(* Logix 5000 AddOnInstructionDefinition export NTEC_MAM; software revision ? *)

TYPE NTEC_Axis :   // NTEC Axis:
STRUCT
   StatDriveCommsOK : BOOL;   // Drive is communicating over ENET IP
   StatServoActionStatus : BOOL;   // Motion is enabled and holding position under power.
   StatDriveWarning : BOOL;   // Drive has a Warning
   StatDriveFault : BOOL;   // Drive is Faulted
   StatMotion_AtTarget : BOOL;   // Motion Target Reached
   StatMotion_FollowingError : BOOL;   // Following Error Fault
   StatMotion_LimitExceeded : BOOL;   // Speed or Position Limit Exceeded
   StatMotion_Halt : BOOL;   // Motor is in Halt, still powered on
   StatQuckStop : BOOL;   // Motor is powered off in Quick Stop
   StatMotion_Homed : BOOL;   // Motion Coordinate System Homed
   StatNewCmdToggle : BOOL;   // Bit toggles after new command accepted
   StatCommandError : BOOL;   // Last Command has an Error
   StatCommandErrorCode : DINT;   // Command Error Code
   StatDriveFaultCode : DINT;   // Drive Fault Code
   StatDriveWarningCode : DINT;   // Drive Warning Code
   StatResettingFault : BOOL;   // In fault reset sequence
   StatReadResponse : DINT;   // Response from a Read CMD
   CMD_IP : BOOL;   // Command is In Process
   CMD_DN : BOOL;   // Command is Done
   CMD_ERR : BOOL;   // Command Error during Comms send to Drive
   PDI_CMD : NTEC_PDI_CMD;   // Commands from AOIs
   PDI_Status : NTEC_PDI_Status;   // Status from Drive out to AOIs
   DriveLimits : NTEC_LimitsInDrive;   // Limits read from Drive
END_STRUCT
END_TYPE

TYPE NTEC_LimitsInDrive :   // These are the limits read from the Drive
STRUCT
   PositionLimitMin : DINT;   // Minimum Allowed Position Target (607Bh:1)
   PositionLimitMax : DINT;   // Maximum Allowed Position Target (607Bh:2)
   SoftPositionLimitMin : DINT;   // Minimum Allowed Position (607Dh:1)
   SoftPositionLimitMax : DINT;   // Minimum Allowed Position (607Dh:2)
   VelocityLimitMin : DINT;   // Maximum Allowed Velocity Target negative direction
   VelocityLimitMax : DINT;   // Maximum Allowed Velocity Target positive direction (607Fh)
   MotorSpeedMin : DINT;   // Maximum motor speed in negative direction
   MotorSpeedMax : DINT;   // Maximum motor speed setting in positive direction (6080h)
   AccelLimitMax : DINT;   // Maximum Allowed Accel Target (60C5h)
   DecelLimitMax : DINT;   // Maximum Allowed Decel Target (60C6h)
   PositionWindowNeg : DINT;   // Position Window - negative direction for At Target (6067h)
   PositionWindowPos : DINT;   // Position Window -positive direction for At Target (+/- this value) (6067h)
   VelocityWindowNeg : DINT;   // Velocity Window - negative side for At Target (+/- this value) (606Dh)
   VelocityWindowPos : DINT;   // Velocity Window - positive side for At Target (+/- this value) (606Dh)
   TorqueMaxNegDir : DINT;   // Maximum Torque Target negative direction (0.1% of motor rated current 2031h) (6072h)
   TorqueMaxPosDir : DINT;   // Maximum Torque Target positive direction (0.1% of motor rated current 2031h) (6072h)
   CurrentMaxNegDir : DINT;   // Maximum Current Target negative direction (in 0.1% of rated setting 2031h) (6073h)
   CurrentMaxPosDir : DINT;   // Maximum Current Target positive direction (in 0.1% of rated setting 2031h) (6073h)
END_STRUCT
END_TYPE

TYPE NTEC_PDI_CMD :   // PDI Command Bytes
STRUCT
   SetValue1 : DINT;
   SetValue2 : INT;
   SetValue3 : SINT;
   CMD : SINT;
   DigitalOutputs : DINT;
   NanoJ_Input1 : DINT;
   Trig : BOOL;   // Trigger the Command
   Halt : BOOL;   // Command a HALT
   QuickStop : BOOL;   // Command a QuickStop
END_STRUCT
END_TYPE

TYPE NTEC_PDI_Status :   // PDI Status Bytes
STRUCT
   Status : INT;
   ErrorCode : INT;
   ReturnValue : DINT;
   PositionActualValue : DINT;
   VelocityActualValue : DINT;
   DigitalInputs : DINT;
   TorqueActualValue : INT;
   AnalogInput1 : INT;
   FollowingError : DINT;
   NanoJ_Output1 : DINT;
END_STRUCT
END_TYPE

ADD_ON_INSTRUCTION NTEC_WRITE   (* revision 1.6, vendor Third Coast Automation, Nashville, TN, ExecutePrescan, ExecuteEnableInFalse *)
// WRITE instruction writes the value entered into the AOI, into the specified object in the Drive.  Enter the target object's index and sub-index (typically 16#xxxx hex values).
// Revision note:
// Release Aug 27, 2024, update CPS instructions LEN
// Help:
// AOI written by:
// Tim Cochran
// Third Coast Automation
// Nashville, TN
// MAS ERR_Codes:
// 2: Input parameter range error – review and fix input parameters.
// 3: Command Error response from the Drive after command sent.
// 10: Communications Failed to Drive.
// 11: Drive Fault during this AOIs command sequence.
// 12: Quick Stop triggered by software outside of this AOI.
// 13: Command Error response from the Drive.
// 14: Enable input changed to False during sequence due to Drive Fault or Offline.
VAR_IN_OUT
   NTEC_Axis : NTEC_Axis; {required}   // NTEC Axis Tag
END_VAR
VAR_INPUT
   Index : DINT; {required}   // Index
   SubIndex : DINT; {required}   // Sub-Index
END_VAR
VAR_OUTPUT
   EN : BOOL; {visible}   // Enabled
   DN : BOOL; {visible}   // Successfully Done
END_VAR
VAR_INPUT
   Value : DINT; {required}   // WriteValue
END_VAR
VAR_OUTPUT
   ERR : BOOL; {visible}   // Instruction Error
   ERR_Code : DINT; {access Read Only, visible}   // Instruction Error Code
END_VAR
VAR
   State : DINT; {access None}
   Enable : BOOL; {access None}
   InputRangesOK : BOOL; {access None}
   local_SubIndex : DINT; {access None}
   local_Index : DINT; {access None}
   tmr_Verify : TIMER; {access None}
   local_Value : DINT; {access None}
END_VAR

ROUTINE EnableInFalse   (* ladder *)
// Enable In False Routine
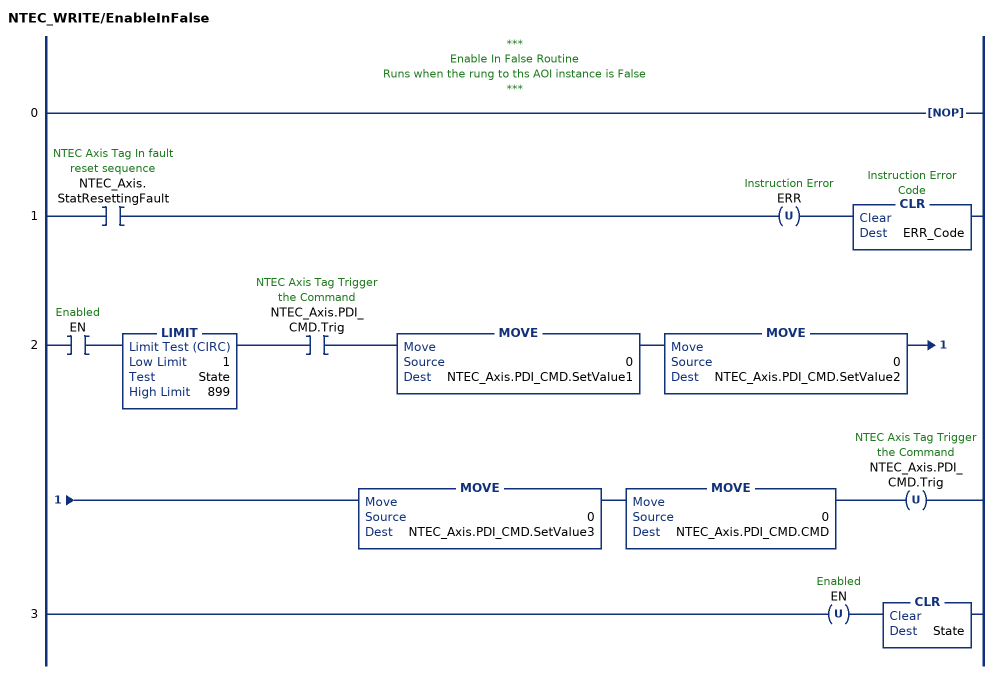
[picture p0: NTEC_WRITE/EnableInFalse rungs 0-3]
   // ***
   // Enable In False Routine
   // Runs when the rung to ths AOI instance is False
   // ***
   0: NOP();
   1: XIC(NTEC_Axis.StatResettingFault)OTU(ERR)CLR(ERR_Code);
   2: XIC(EN)LIMIT(1,State,899)XIC(NTEC_Axis.PDI_CMD.Trig)MOVE(0,NTEC_Axis.PDI_CMD.SetValue1)MOVE(0,NTEC_Axis.PDI_CMD.SetValue2)MOVE(0,NTEC_Axis.PDI_CMD.SetValue3)MOVE(0,NTEC_Axis.PDI_CMD.CMD)OTU(NTEC_Axis.PDI_CMD.Trig);
   3: OTU(EN)CLR(State);
END_ROUTINE

ROUTINE Logic   (* ladder *)
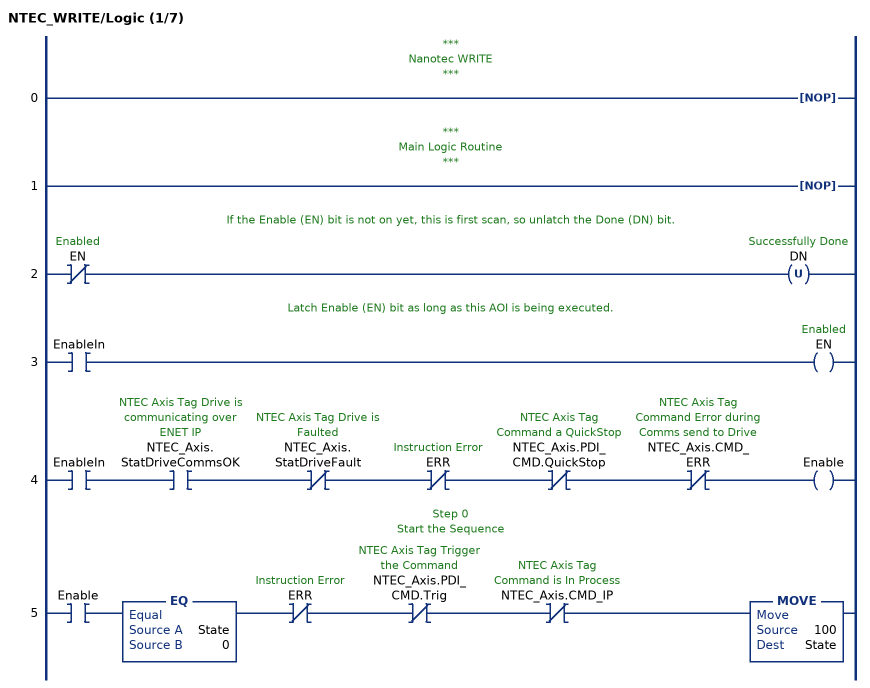
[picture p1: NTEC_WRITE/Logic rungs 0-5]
   // ***
   // Nanotec WRITE
   // ***
   0: NOP();
   // ***
   // Main Logic Routine
   // ***
   1: NOP();
   // If the Enable (EN) bit is not on yet, this is first scan, so unlatch the Done (DN) bit.
   2: XIO(EN)OTU(DN);
   // Latch Enable (EN) bit as long as this AOI is being executed.
   3: XIC(EnableIn)OTE(EN);
   4: XIC(EnableIn)XIC(NTEC_Axis.StatDriveCommsOK)XIO(NTEC_Axis.StatDriveFault)XIO(ERR)XIO(NTEC_Axis.PDI_CMD.QuickStop)XIO(NTEC_Axis.CMD_ERR)OTE(Enable);
   // Step 0
   // Start the Sequence
   5: XIC(Enable)EQ(State,0)XIO(ERR)XIO(NTEC_Axis.PDI_CMD.Trig)XIO(NTEC_Axis.CMD_IP)MOVE(100,State);
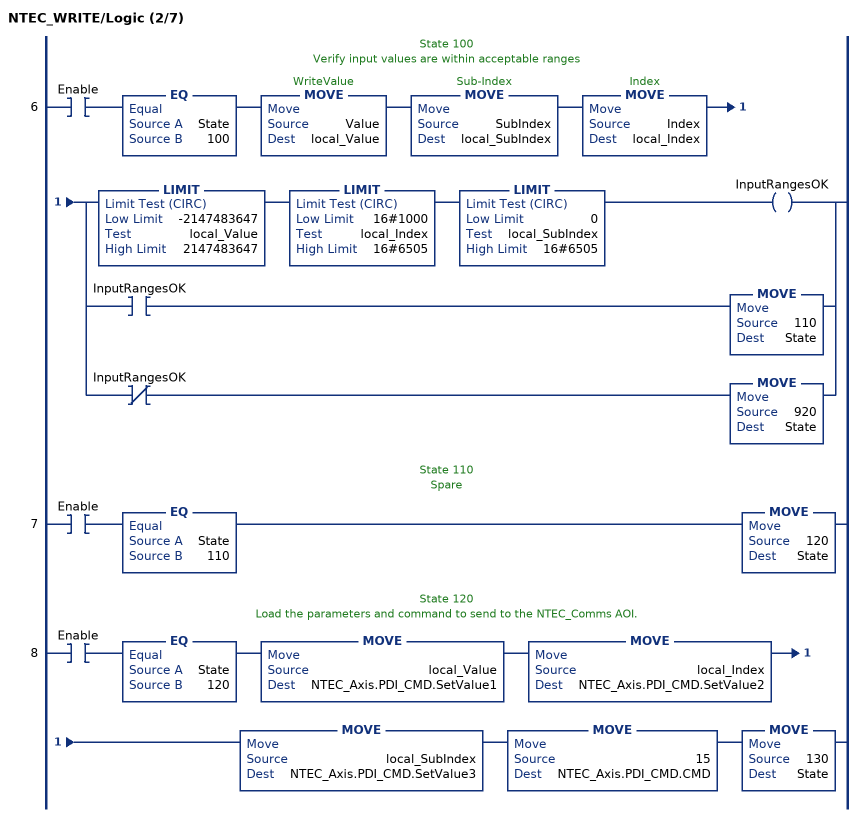
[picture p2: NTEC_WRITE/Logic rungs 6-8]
   // State 100
   // Verify input values are within acceptable ranges
   6: XIC(Enable)EQ(State,100)MOVE(Value,local_Value)MOVE(SubIndex,local_SubIndex)MOVE(Index,local_Index)[LIMIT(-2147483647,local_Value,2147483647) LIMIT(16#1000,local_Index,16#6505) LIMIT(0,local_SubIndex,16#6505) OTE(InputRangesOK) ,XIC(InputRangesOK) MOVE(110,State) ,XIO(InputRangesOK) MOVE(920,State) ];
   // State 110
   // Spare
   7: XIC(Enable)EQ(State,110)MOVE(120,State);
   // State 120
   // Load the parameters and command to send to the NTEC_Comms AOI.
   8: XIC(Enable)EQ(State,120)MOVE(local_Value,NTEC_Axis.PDI_CMD.SetValue1)MOVE(local_Index,NTEC_Axis.PDI_CMD.SetValue2)MOVE(local_SubIndex,NTEC_Axis.PDI_CMD.SetValue3)MOVE(15,NTEC_Axis.PDI_CMD.CMD)MOVE(130,State);
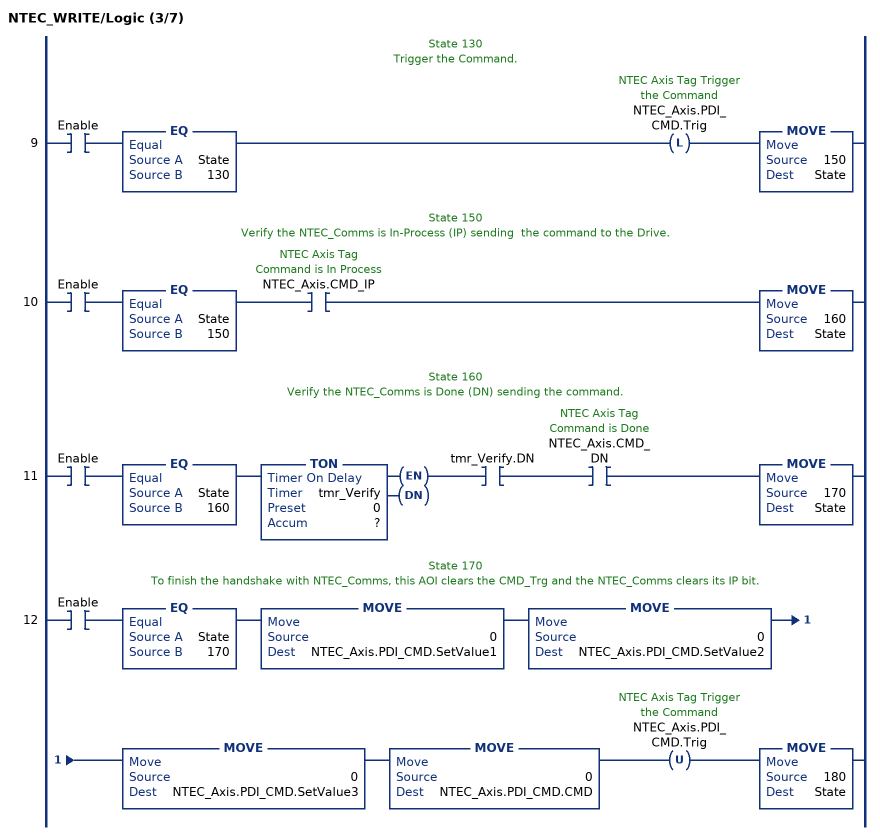
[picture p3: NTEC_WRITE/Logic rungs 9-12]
   // State 130
   // Trigger the Command.
   9: XIC(Enable)EQ(State,130)OTL(NTEC_Axis.PDI_CMD.Trig)MOVE(150,State);
   // State 150
   // Verify the NTEC_Comms is In-Process (IP) sending  the command to the Drive.
   10: XIC(Enable)EQ(State,150)XIC(NTEC_Axis.CMD_IP)MOVE(160,State);
   // State 160
   // Verify the NTEC_Comms is Done (DN) sending the command.
   11: XIC(Enable)EQ(State,160)TON(tmr_Verify,?,?)XIC(tmr_Verify.DN)XIC(NTEC_Axis.CMD_DN)MOVE(170,State);
   // State 170
   // To finish the handshake with NTEC_Comms, this AOI clears the CMD_Trg and the NTEC_Comms clears its IP bit.
   12: XIC(Enable)EQ(State,170)MOVE(0,NTEC_Axis.PDI_CMD.SetValue1)MOVE(0,NTEC_Axis.PDI_CMD.SetValue2)MOVE(0,NTEC_Axis.PDI_CMD.SetValue3)MOVE(0,NTEC_Axis.PDI_CMD.CMD)OTU(NTEC_Axis.PDI_CMD.Trig)MOVE(180,State);
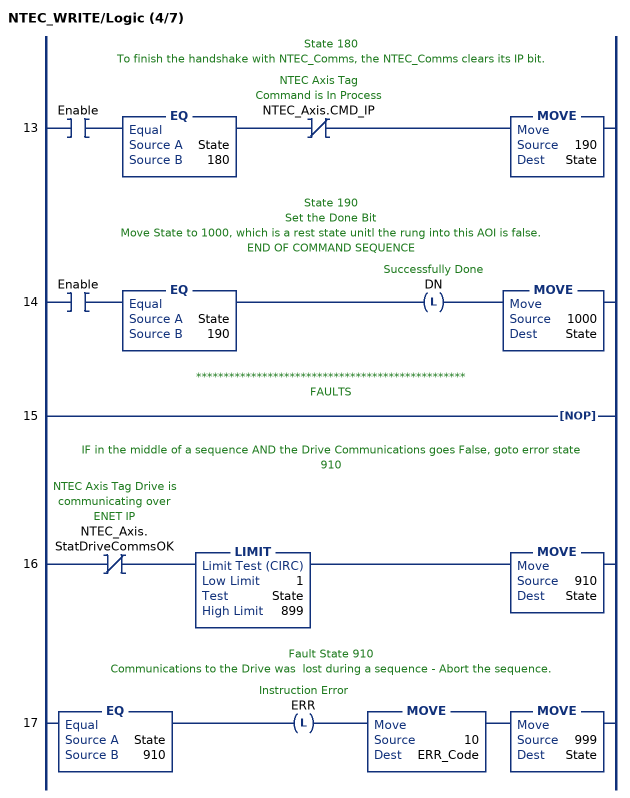
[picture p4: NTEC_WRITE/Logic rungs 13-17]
   // State 180
   // To finish the handshake with NTEC_Comms, the NTEC_Comms clears its IP bit.
   13: XIC(Enable)EQ(State,180)XIO(NTEC_Axis.CMD_IP)MOVE(190,State);
   // State 190
   // Set the Done Bit
   // Move State to 1000, which is a rest state unitl the rung into this AOI is false.
   // END OF COMMAND SEQUENCE
   14: XIC(Enable)EQ(State,190)OTL(DN)MOVE(1000,State);
   // *************************************************
   // FAULTS
   15: NOP();
   // IF in the middle of a sequence AND the Drive Communications goes False, goto error state 910
   16: XIO(NTEC_Axis.StatDriveCommsOK)LIMIT(1,State,899)MOVE(910,State);
   // Fault State 910
   // Communications to the Drive was  lost during a sequence - Abort the sequence.
   17: EQ(State,910)OTL(ERR)MOVE(10,ERR_Code)MOVE(999,State);
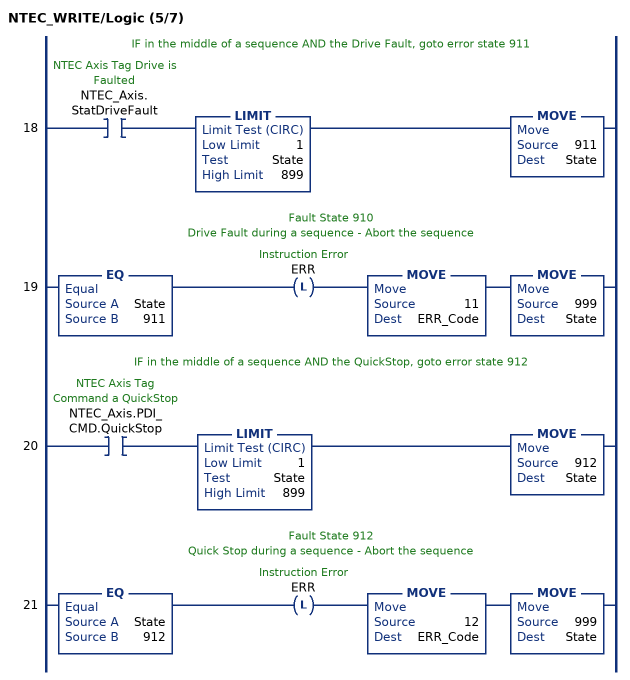
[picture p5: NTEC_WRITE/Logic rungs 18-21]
   // IF in the middle of a sequence AND the Drive Fault, goto error state 911
   18: XIC(NTEC_Axis.StatDriveFault)LIMIT(1,State,899)MOVE(911,State);
   // Fault State 910
   // Drive Fault during a sequence - Abort the sequence
   19: EQ(State,911)OTL(ERR)MOVE(11,ERR_Code)MOVE(999,State);
   // IF in the middle of a sequence AND the QuickStop, goto error state 912
   20: XIC(NTEC_Axis.PDI_CMD.QuickStop)LIMIT(1,State,899)MOVE(912,State);
   // Fault State 912
   // Quick Stop during a sequence - Abort the sequence
   21: EQ(State,912)OTL(ERR)MOVE(12,ERR_Code)MOVE(999,State);
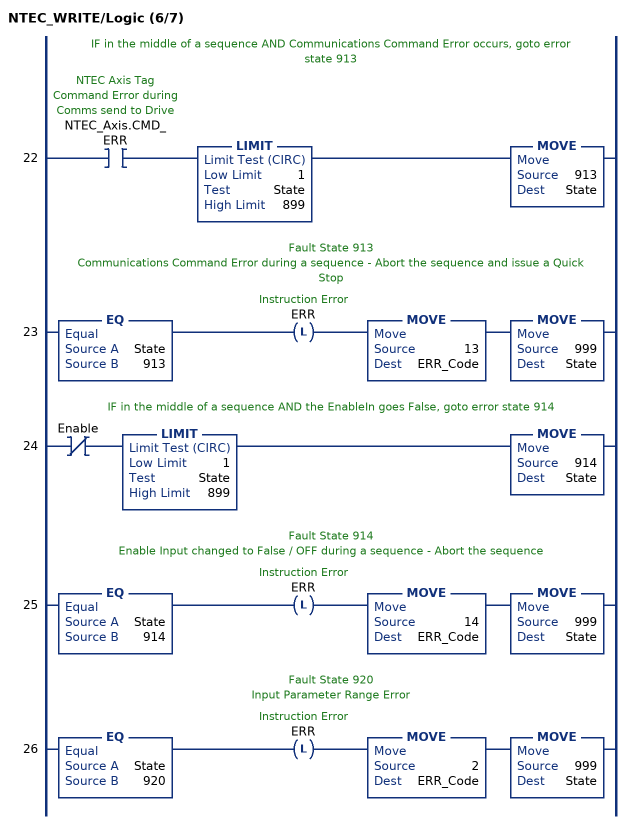
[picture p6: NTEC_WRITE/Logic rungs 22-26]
   // IF in the middle of a sequence AND Communications Command Error occurs, goto error state 913
   22: XIC(NTEC_Axis.CMD_ERR)LIMIT(1,State,899)MOVE(913,State);
   // Fault State 913
   // Communications Command Error during a sequence - Abort the sequence and issue a Quick Stop
   23: EQ(State,913)OTL(ERR)MOVE(13,ERR_Code)MOVE(999,State);
   // IF in the middle of a sequence AND the EnableIn goes False, goto error state 914
   24: XIO(Enable)LIMIT(1,State,899)MOVE(914,State);
   // Fault State 914
   // Enable Input changed to False / OFF during a sequence - Abort the sequence
   25: EQ(State,914)OTL(ERR)MOVE(14,ERR_Code)MOVE(999,State);
   // Fault State 920
   // Input Parameter Range Error
   26: EQ(State,920)OTL(ERR)MOVE(2,ERR_Code)MOVE(999,State);
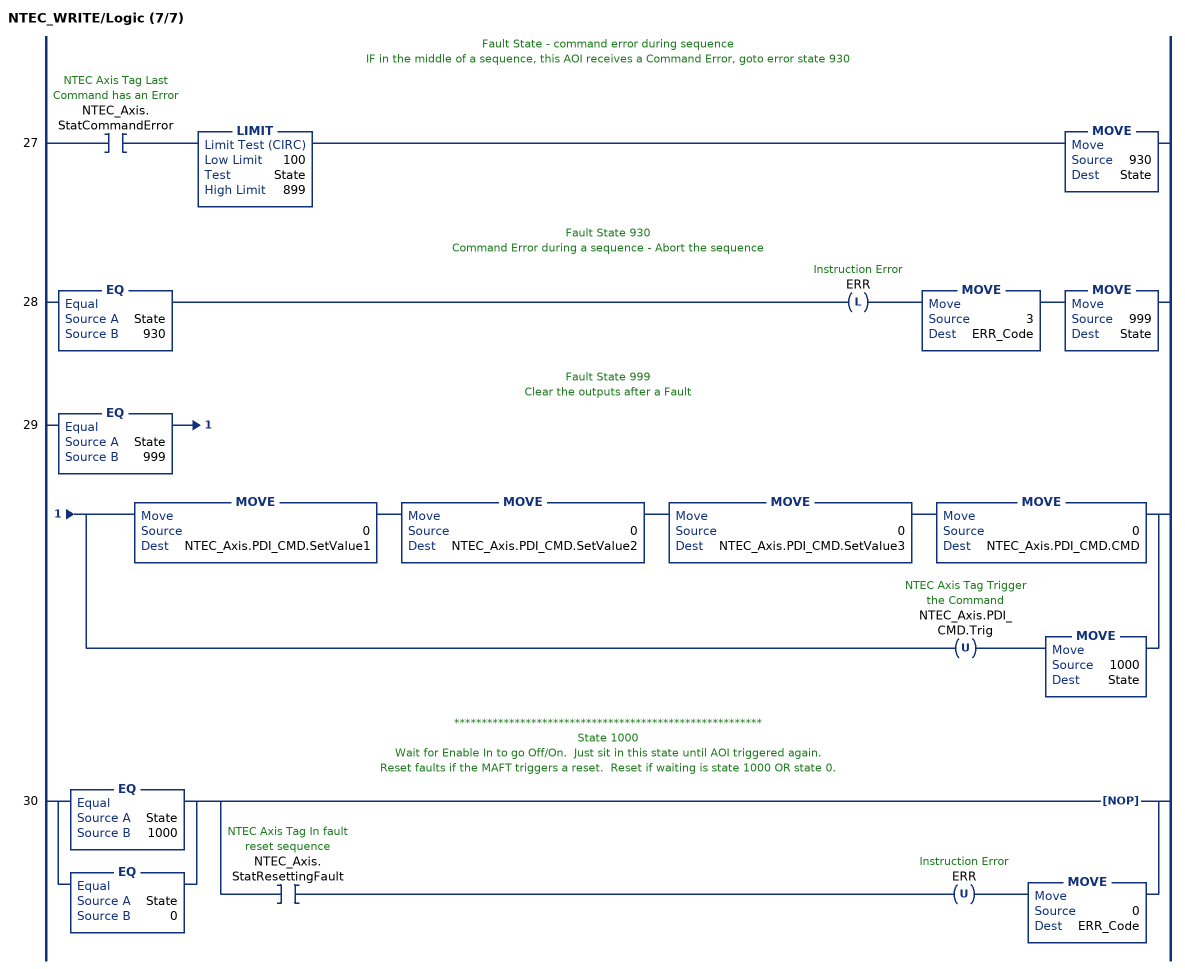
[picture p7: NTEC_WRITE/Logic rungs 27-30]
   // Fault State - command error during sequence
   // IF in the middle of a sequence, this AOI receives a Command Error, goto error state 930
   27: XIC(NTEC_Axis.StatCommandError)LIMIT(100,State,899)MOVE(930,State);
   // Fault State 930
   // Command Error during a sequence - Abort the sequence
   28: EQ(State,930)OTL(ERR)MOVE(3,ERR_Code)MOVE(999,State);
   // Fault State 999
   // Clear the outputs after a Fault
   29: EQ(State,999)[MOVE(0,NTEC_Axis.PDI_CMD.SetValue1) MOVE(0,NTEC_Axis.PDI_CMD.SetValue2) MOVE(0,NTEC_Axis.PDI_CMD.SetValue3) MOVE(0,NTEC_Axis.PDI_CMD.CMD) ,OTU(NTEC_Axis.PDI_CMD.Trig) MOVE(1000,State) ];
   // ********************************************************
   // State 1000
   // Wait for Enable In to go Off/On.  Just sit in this state until AOI triggered again.
   // Reset faults if the MAFT triggers a reset.  Reset if waiting is state 1000 OR state 0.
   30: [EQ(State,1000) ,EQ(State,0) ][NOP() ,XIC(NTEC_Axis.StatResettingFault) OTU(ERR) MOVE(0,ERR_Code) ];
END_ROUTINE

ROUTINE Postscan   (* ladder *)
// Home Post-Scan Routine
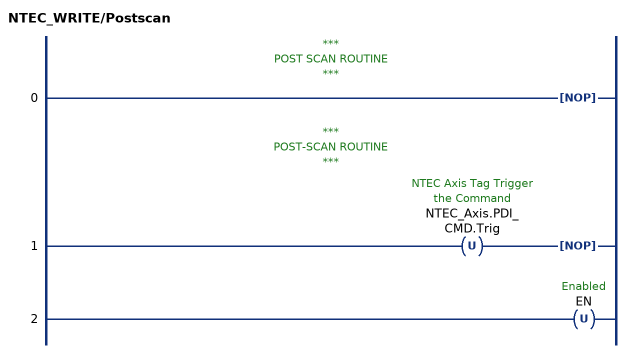
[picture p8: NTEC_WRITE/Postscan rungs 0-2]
   // ***
   // POST SCAN ROUTINE
   // ***
   0: NOP();
   // ***
   // POST-SCAN ROUTINE
   // ***
   1: OTU(NTEC_Axis.PDI_CMD.Trig)NOP();
   2: OTU(EN);
END_ROUTINE

ROUTINE Prescan   (* ladder *)
// Home Pre-Scan Routine
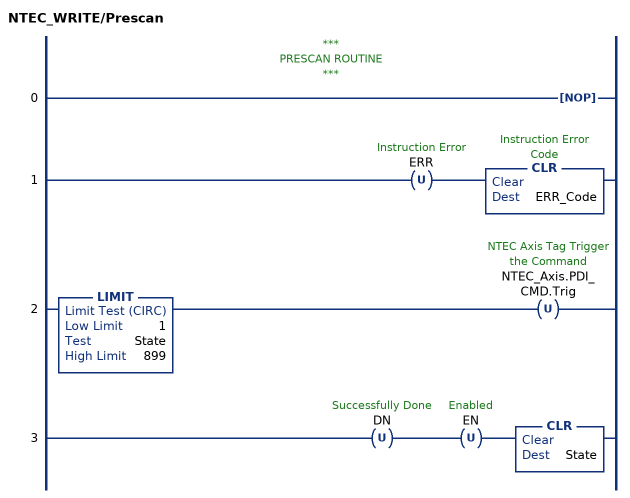
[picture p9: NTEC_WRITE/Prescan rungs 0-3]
   // ***
   // PRESCAN ROUTINE
   // ***
   0: NOP();
   1: OTU(ERR)CLR(ERR_Code);
   2: LIMIT(1,State,899)OTU(NTEC_Axis.PDI_CMD.Trig);
   3: OTU(DN)OTU(EN)CLR(State);
END_ROUTINE
END_ADD_ON_INSTRUCTION

ADD_ON_INSTRUCTION NTEC_MAM   (* revision 1.6, vendor Third Coast Automation, Nashville, TN, ExecutePrescan, ExecuteEnableInFalse *)
// Motion Axis Move (MAM)
// Move the servo axis to a target position.
// Move Type:
// 1=Absolute
// 2=Incremental (Relative)
// All input parameters are entered into the AOI in whole numbers, in the units as setup and scaled in the Drive.
// Revision note:
// Release Aug 27, 2024, update CPS instructions LEN
// Help:
// AOI written by:
// Tim Cochran
// Third Coast Automation
// Nashville, TN
// MAM ERR_Codes:
// 2: Input parameter range error – review and fix input parameters.
// 3: Command Error response from the Drive after command sent.
// 4: Command Error after Accel value was sent to the Drive.
// 5: Command Error after Decel value was sent to the Drive.
// 10: Communications Failed to Drive.
// 11: Drive Fault during this AOIs command sequence.
// 12: Quick Stop triggered by software outside of this AOI.
// 13: Command Error response from the Drive.
// 14: Enable input changed to False during sequence due to Drive Fault or Offline.
VAR_IN_OUT
   NTEC_Axis : NTEC_Axis; {required}   // NTEC Axis Tag
END_VAR
VAR_INPUT
   MoveType : DINT; {required}   // 1=Absolute 2= Relative (Incremental)
   Position : DINT; {required}   // Position value for move location
   Velocity : DINT; {required}   // Velocity in Drive units / sec
   Acceleration : DINT; {required}   // Accel in Drive units/sec^2
   Deceleration : DINT; {required}   // Decel in Drive units/sec^2
END_VAR
VAR_OUTPUT
   EN : BOOL; {access Read Only, visible}   // Enabled
   IP : BOOL; {visible}   // In Process
   DN : BOOL; {visible}   // Successfully Done
   ERR : BOOL; {visible}   // Instruction Error
   ERR_Code : DINT; {access Read Only, visible}   // Instruction Error Code
END_VAR
VAR
   State : DINT; {access None}
   Enable : BOOL; {access None}
   local_MoveType : DINT := 2; {access None}
   local_Position : DINT; {access None}
   local_Acceleration : DINT; {access None}
   InputRangesOK : BOOL; {access None}
   tmr_Verify : TIMER := (PRE := 20); {access None}
   local_Deceleration : DINT; {access None}
   local_Velocity : INT; {access None}
   Write1_cntrl : NTEC_WRITE; {access None}
   Write2_cntrl : NTEC_WRITE; {access None}
   MoveStarted : BOOL; {access None}
   MovePositionDelta : DINT; {access None}
   LowLimitPositionWindow : DINT := -50; {access None}
   HighLimitPositionWindow : DINT := 50; {access None}
END_VAR

ROUTINE EnableInFalse   (* ladder *)
// Enable In False Routine
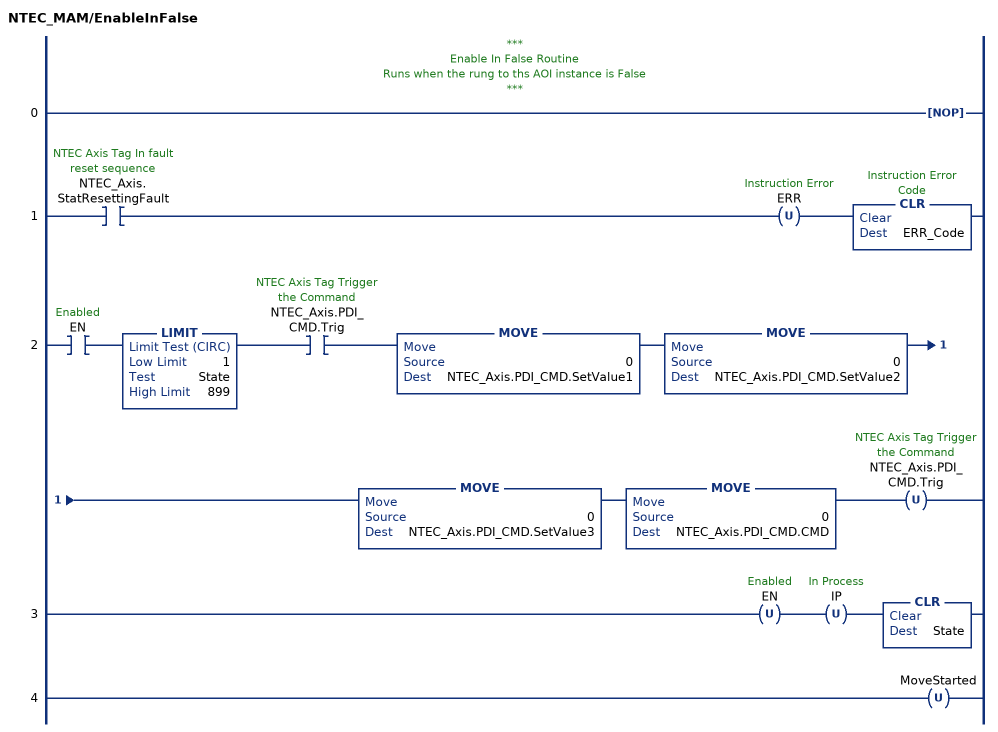
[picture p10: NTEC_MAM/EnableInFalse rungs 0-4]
   // ***
   // Enable In False Routine
   // Runs when the rung to ths AOI instance is False
   // ***
   0: NOP();
   1: XIC(NTEC_Axis.StatResettingFault)OTU(ERR)CLR(ERR_Code);
   2: XIC(EN)LIMIT(1,State,899)XIC(NTEC_Axis.PDI_CMD.Trig)MOVE(0,NTEC_Axis.PDI_CMD.SetValue1)MOVE(0,NTEC_Axis.PDI_CMD.SetValue2)MOVE(0,NTEC_Axis.PDI_CMD.SetValue3)MOVE(0,NTEC_Axis.PDI_CMD.CMD)OTU(NTEC_Axis.PDI_CMD.Trig);
   3: OTU(EN)OTU(IP)CLR(State);
   4: OTU(MoveStarted);
END_ROUTINE

ROUTINE Logic   (* ladder *)
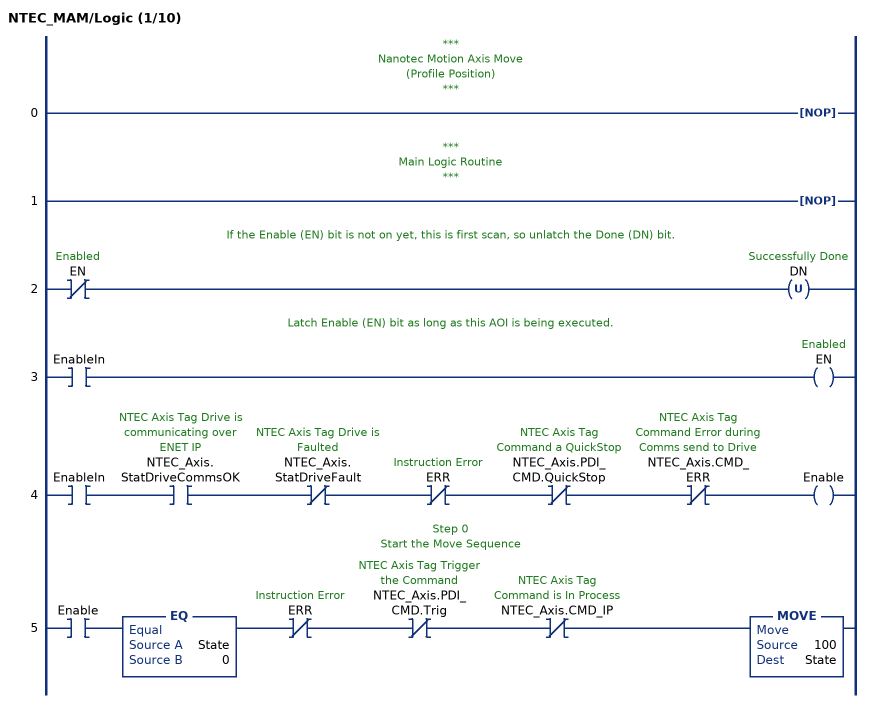
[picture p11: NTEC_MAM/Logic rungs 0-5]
   // ***
   // Nanotec Motion Axis Move
   // (Profile Position)
   // ***
   0: NOP();
   // ***
   // Main Logic Routine
   // ***
   1: NOP();
   // If the Enable (EN) bit is not on yet, this is first scan, so unlatch the Done (DN) bit.
   2: XIO(EN)OTU(DN);
   // Latch Enable (EN) bit as long as this AOI is being executed.
   3: XIC(EnableIn)OTE(EN);
   4: XIC(EnableIn)XIC(NTEC_Axis.StatDriveCommsOK)XIO(NTEC_Axis.StatDriveFault)XIO(ERR)XIO(NTEC_Axis.PDI_CMD.QuickStop)XIO(NTEC_Axis.CMD_ERR)OTE(Enable);
   // Step 0
   // Start the Move Sequence
   5: XIC(Enable)EQ(State,0)XIO(ERR)XIO(NTEC_Axis.PDI_CMD.Trig)XIO(NTEC_Axis.CMD_IP)MOVE(100,State);
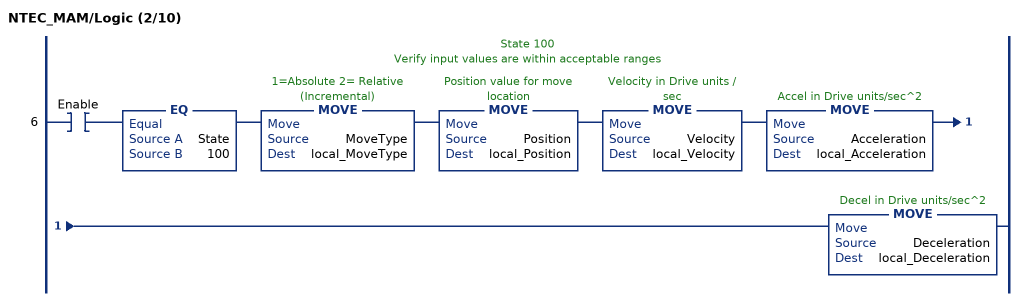
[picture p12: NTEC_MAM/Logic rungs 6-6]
   // State 100
   // Verify input values are within acceptable ranges
   6: XIC(Enable)EQ(State,100)MOVE(MoveType,local_MoveType)MOVE(Position,local_Position)MOVE(Velocity,local_Velocity)MOVE(Acceleration,local_Acceleration)MOVE(Deceleration,local_Deceleration);
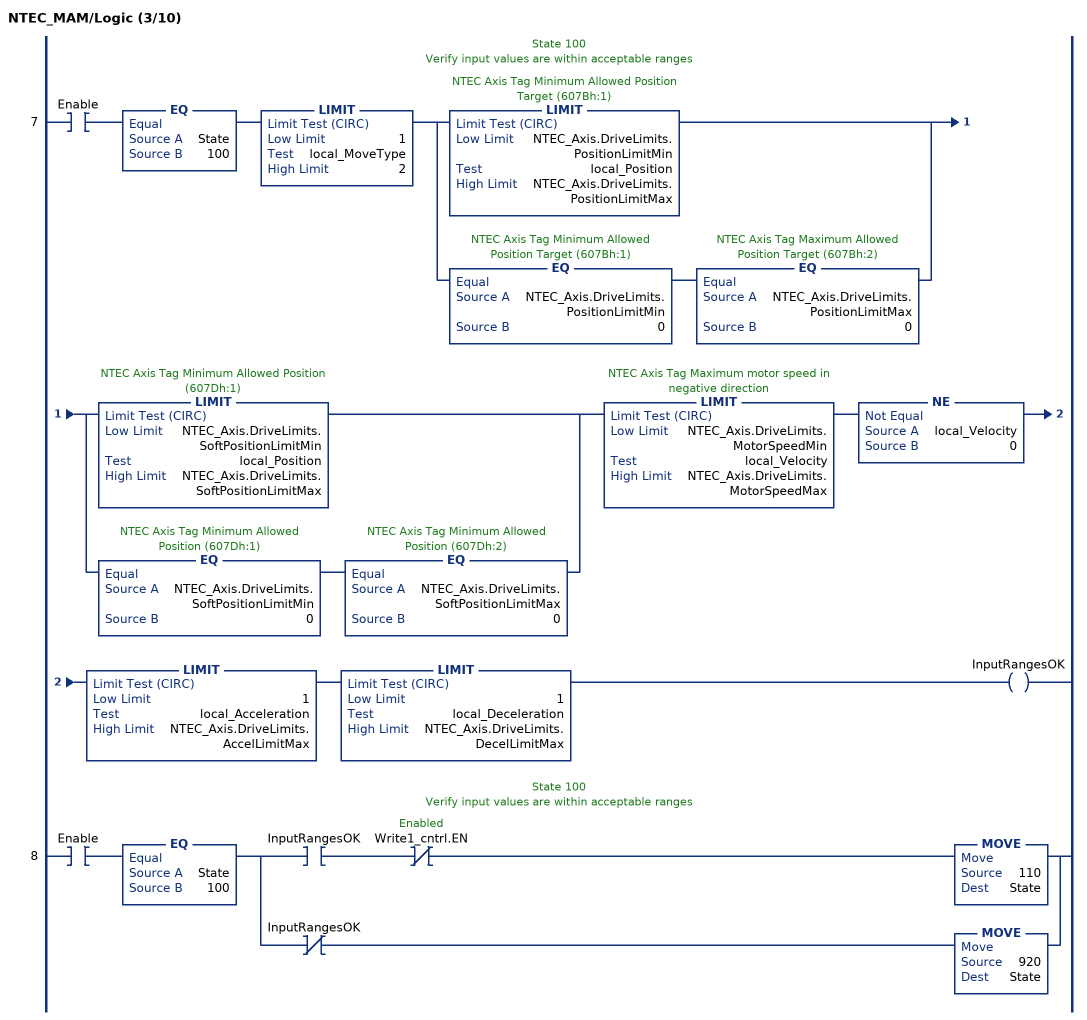
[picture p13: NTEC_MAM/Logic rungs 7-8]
   // State 100
   // Verify input values are within acceptable ranges
   7: XIC(Enable)EQ(State,100)LIMIT(1,local_MoveType,2)[LIMIT(NTEC_Axis.DriveLimits.PositionLimitMin,local_Position,NTEC_Axis.DriveLimits.PositionLimitMax) ,EQ(NTEC_Axis.DriveLimits.PositionLimitMin,0) EQ(NTEC_Axis.DriveLimits.PositionLimitMax,0) ][LIMIT(NTEC_Axis.DriveLimits.SoftPositionLimitMin,local_Position,NTEC_Axis.DriveLimits.SoftPositionLimitMax) ,EQ(NTEC_Axis.DriveLimits.SoftPositionLimitMin,0) EQ(NTEC_Axis.DriveLimits.SoftPositionLimitMax,0) ]LIMIT(NTEC_Axis.DriveLimits.MotorSpeedMin,local_Velocity,NTEC_Axis.DriveLimits.MotorSpeedMax)NE(local_Velocity,0)LIMIT(1,local_Acceleration,NTEC_Axis.DriveLimits.AccelLimitMax)LIMIT(1,local_Deceleration,NTEC_Axis.DriveLimits.DecelLimitMax)OTE(InputRangesOK);
   // State 100
   // Verify input values are within acceptable ranges
   8: XIC(Enable)EQ(State,100)[XIC(InputRangesOK) XIO(Write1_cntrl.EN) MOVE(110,State) ,XIO(InputRangesOK) MOVE(920,State) ];
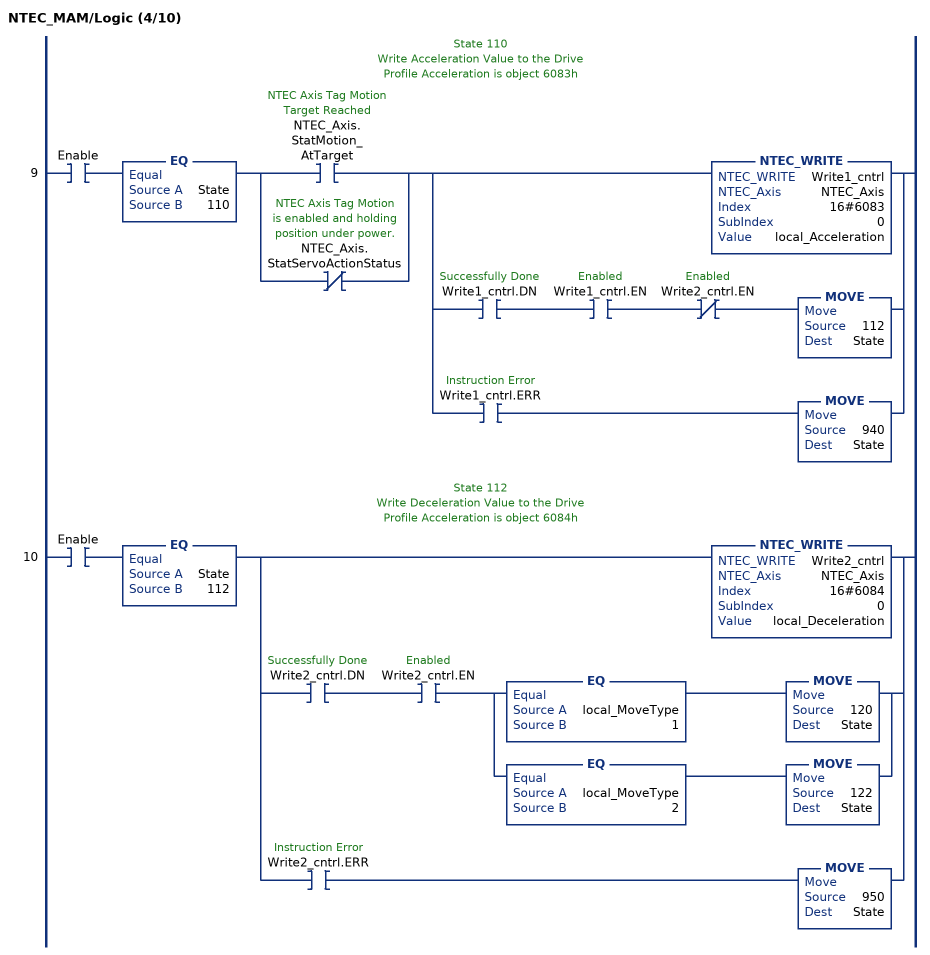
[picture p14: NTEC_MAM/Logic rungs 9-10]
   // State 110
   // Write Acceleration Value to the Drive
   // Profile Acceleration is object 6083h
   9: XIC(Enable)EQ(State,110)[XIC(NTEC_Axis.StatMotion_AtTarget) ,XIO(NTEC_Axis.StatServoActionStatus) ][NTEC_WRITE(Write1_cntrl,NTEC_Axis,16#6083,0,local_Acceleration) ,XIC(Write1_cntrl.DN) XIC(Write1_cntrl.EN) XIO(Write2_cntrl.EN) MOVE(112,State) ,XIC(Write1_cntrl.ERR) MOVE(940,State) ];
   // State 112
   // Write Deceleration Value to the Drive
   // Profile Acceleration is object 6084h
   10: XIC(Enable)EQ(State,112)[NTEC_WRITE(Write2_cntrl,NTEC_Axis,16#6084,0,local_Deceleration) ,XIC(Write2_cntrl.DN) XIC(Write2_cntrl.EN) [EQ(local_MoveType,1) MOVE(120,State) ,EQ(local_MoveType,2) MOVE(122,State) ] ,XIC(Write2_cntrl.ERR) MOVE(950,State) ];
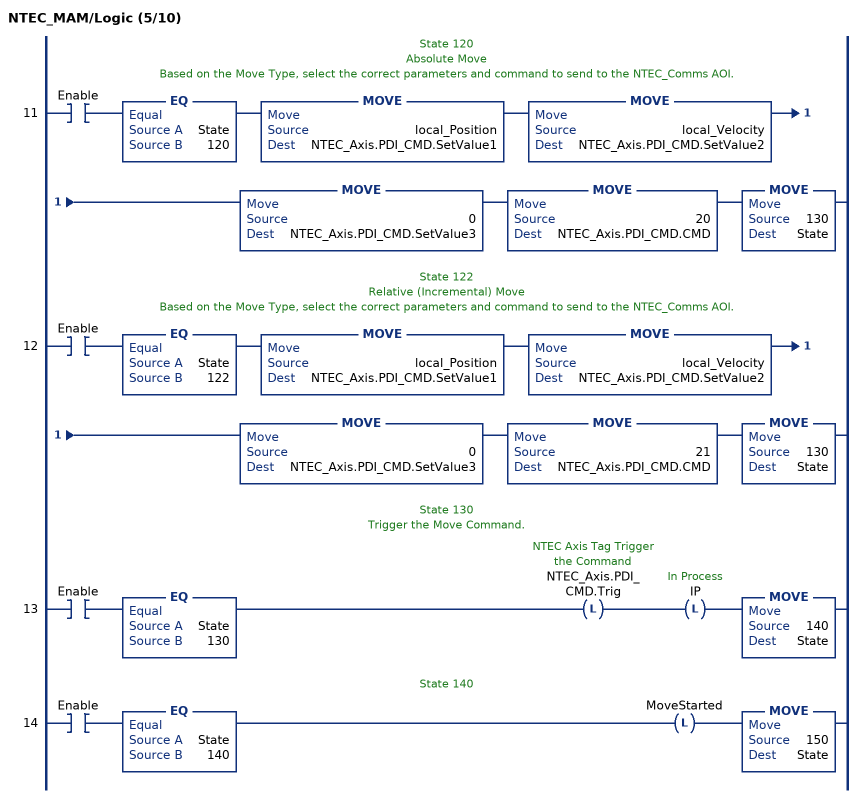
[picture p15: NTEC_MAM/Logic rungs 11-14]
   // State 120
   // Absolute Move
   // Based on the Move Type, select the correct parameters and command to send to the NTEC_Comms AOI.
   11: XIC(Enable)EQ(State,120)MOVE(local_Position,NTEC_Axis.PDI_CMD.SetValue1)MOVE(local_Velocity,NTEC_Axis.PDI_CMD.SetValue2)MOVE(0,NTEC_Axis.PDI_CMD.SetValue3)MOVE(20,NTEC_Axis.PDI_CMD.CMD)MOVE(130,State);
   // State 122
   // Relative (Incremental) Move
   // Based on the Move Type, select the correct parameters and command to send to the NTEC_Comms AOI.
   12: XIC(Enable)EQ(State,122)MOVE(local_Position,NTEC_Axis.PDI_CMD.SetValue1)MOVE(local_Velocity,NTEC_Axis.PDI_CMD.SetValue2)MOVE(0,NTEC_Axis.PDI_CMD.SetValue3)MOVE(21,NTEC_Axis.PDI_CMD.CMD)MOVE(130,State);
   // State 130
   // Trigger the Move Command.
   13: XIC(Enable)EQ(State,130)OTL(NTEC_Axis.PDI_CMD.Trig)OTL(IP)MOVE(140,State);
   // State 140
   14: XIC(Enable)EQ(State,140)OTL(MoveStarted)MOVE(150,State);
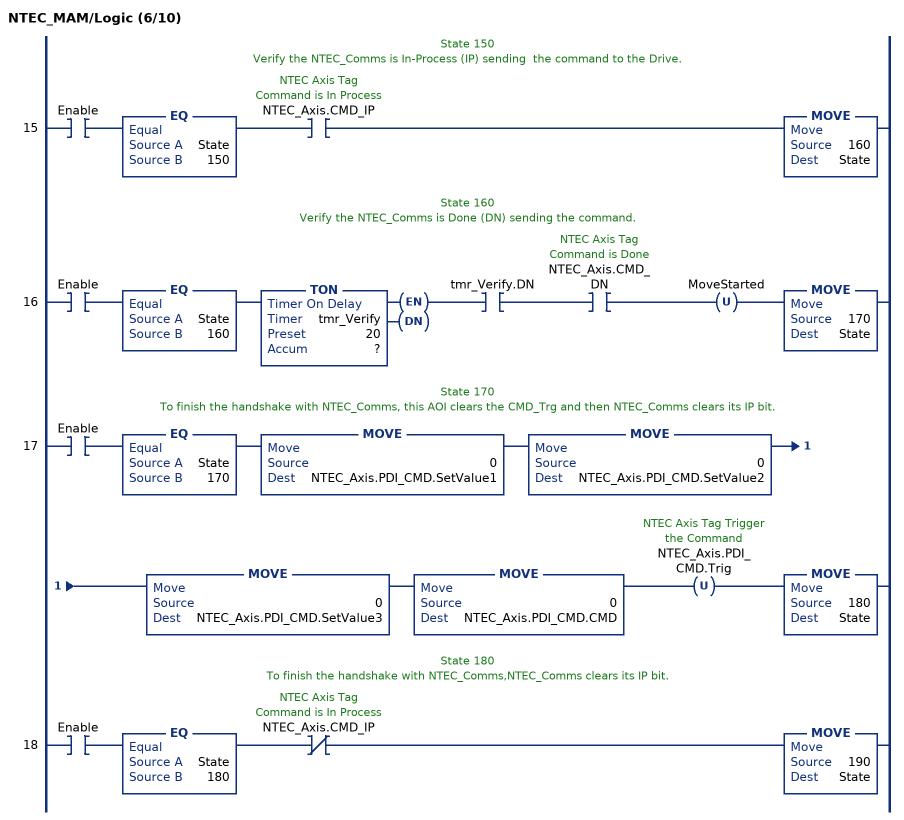
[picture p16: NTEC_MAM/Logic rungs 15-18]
   // State 150
   // Verify the NTEC_Comms is In-Process (IP) sending  the command to the Drive.
   15: XIC(Enable)EQ(State,150)XIC(NTEC_Axis.CMD_IP)MOVE(160,State);
   // State 160
   // Verify the NTEC_Comms is Done (DN) sending the command.
   16: XIC(Enable)EQ(State,160)TON(tmr_Verify,?,?)XIC(tmr_Verify.DN)XIC(NTEC_Axis.CMD_DN)OTU(MoveStarted)MOVE(170,State);
   // State 170
   // To finish the handshake with NTEC_Comms, this AOI clears the CMD_Trg and then NTEC_Comms clears its IP bit.
   17: XIC(Enable)EQ(State,170)MOVE(0,NTEC_Axis.PDI_CMD.SetValue1)MOVE(0,NTEC_Axis.PDI_CMD.SetValue2)MOVE(0,NTEC_Axis.PDI_CMD.SetValue3)MOVE(0,NTEC_Axis.PDI_CMD.CMD)OTU(NTEC_Axis.PDI_CMD.Trig)MOVE(180,State);
   // State 180
   // To finish the handshake with NTEC_Comms,NTEC_Comms clears its IP bit.
   18: XIC(Enable)EQ(State,180)XIO(NTEC_Axis.CMD_IP)MOVE(190,State);
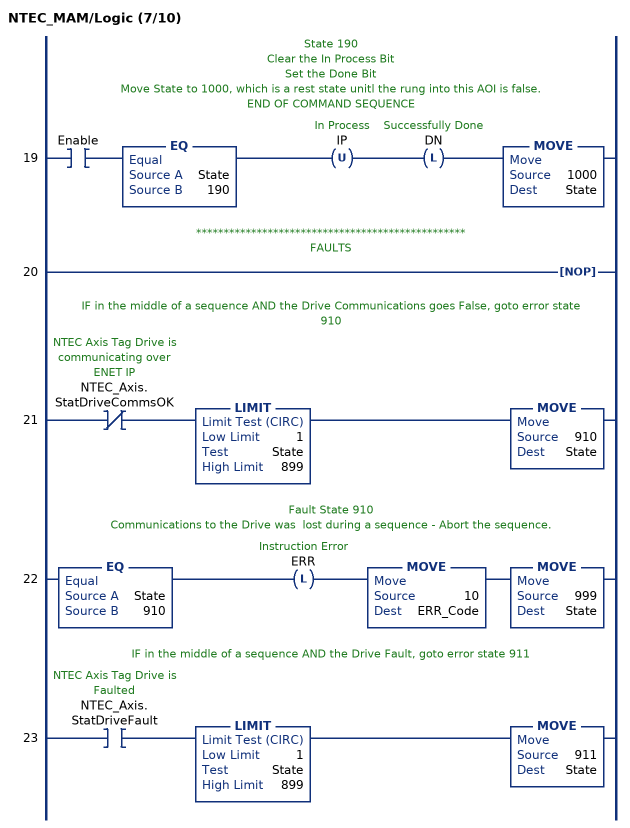
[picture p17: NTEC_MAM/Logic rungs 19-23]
   // State 190
   // Clear the In Process Bit
   // Set the Done Bit
   // Move State to 1000, which is a rest state unitl the rung into this AOI is false.
   // END OF COMMAND SEQUENCE
   19: XIC(Enable)EQ(State,190)OTU(IP)OTL(DN)MOVE(1000,State);
   // *************************************************
   // FAULTS
   20: NOP();
   // IF in the middle of a sequence AND the Drive Communications goes False, goto error state 910
   21: XIO(NTEC_Axis.StatDriveCommsOK)LIMIT(1,State,899)MOVE(910,State);
   // Fault State 910
   // Communications to the Drive was  lost during a sequence - Abort the sequence.
   22: EQ(State,910)OTL(ERR)MOVE(10,ERR_Code)MOVE(999,State);
   // IF in the middle of a sequence AND the Drive Fault, goto error state 911
   23: XIC(NTEC_Axis.StatDriveFault)LIMIT(1,State,899)MOVE(911,State);
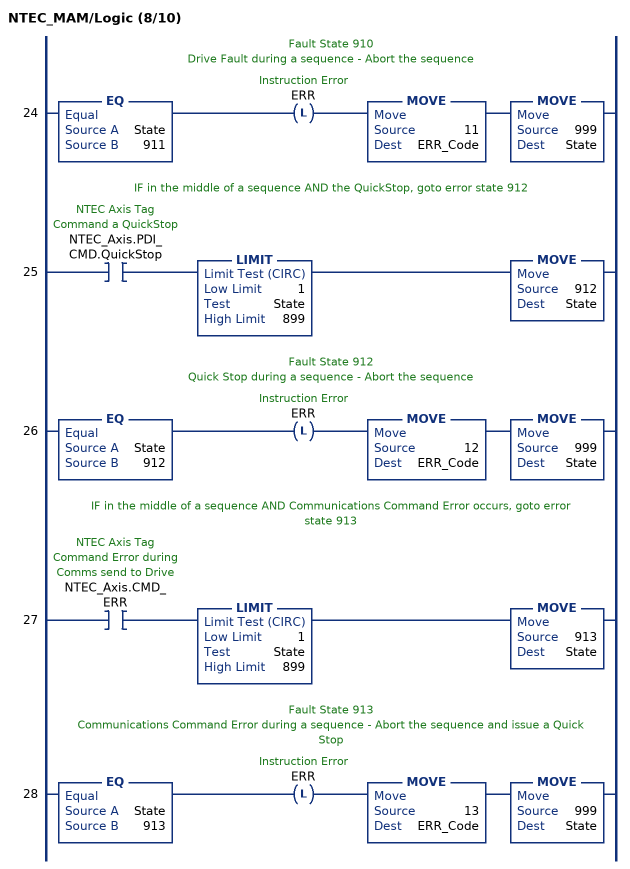
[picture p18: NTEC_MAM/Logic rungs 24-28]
   // Fault State 910
   // Drive Fault during a sequence - Abort the sequence
   24: EQ(State,911)OTL(ERR)MOVE(11,ERR_Code)MOVE(999,State);
   // IF in the middle of a sequence AND the QuickStop, goto error state 912
   25: XIC(NTEC_Axis.PDI_CMD.QuickStop)LIMIT(1,State,899)MOVE(912,State);
   // Fault State 912
   // Quick Stop during a sequence - Abort the sequence
   26: EQ(State,912)OTL(ERR)MOVE(12,ERR_Code)MOVE(999,State);
   // IF in the middle of a sequence AND Communications Command Error occurs, goto error state 913
   27: XIC(NTEC_Axis.CMD_ERR)LIMIT(1,State,899)MOVE(913,State);
   // Fault State 913
   // Communications Command Error during a sequence - Abort the sequence and issue a Quick Stop
   28: EQ(State,913)OTL(ERR)MOVE(13,ERR_Code)MOVE(999,State);
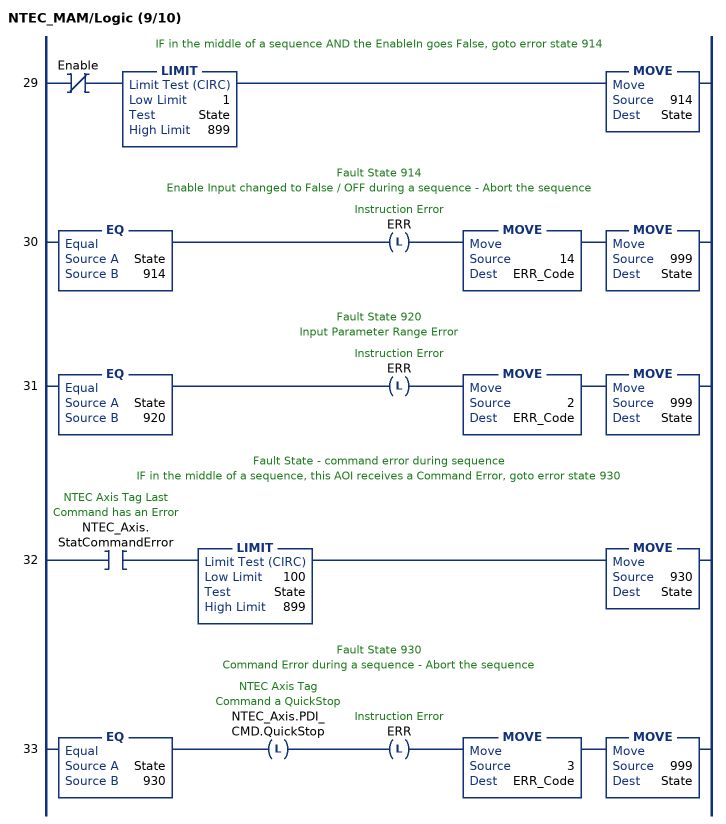
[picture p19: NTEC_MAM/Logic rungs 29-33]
   // IF in the middle of a sequence AND the EnableIn goes False, goto error state 914
   29: XIO(Enable)LIMIT(1,State,899)MOVE(914,State);
   // Fault State 914
   // Enable Input changed to False / OFF during a sequence - Abort the sequence
   30: EQ(State,914)OTL(ERR)MOVE(14,ERR_Code)MOVE(999,State);
   // Fault State 920
   // Input Parameter Range Error
   31: EQ(State,920)OTL(ERR)MOVE(2,ERR_Code)MOVE(999,State);
   // Fault State - command error during sequence
   // IF in the middle of a sequence, this AOI receives a Command Error, goto error state 930
   32: XIC(NTEC_Axis.StatCommandError)LIMIT(100,State,899)MOVE(930,State);
   // Fault State 930
   // Command Error during a sequence - Abort the sequence
   33: EQ(State,930)OTL(NTEC_Axis.PDI_CMD.QuickStop)OTL(ERR)MOVE(3,ERR_Code)MOVE(999,State);
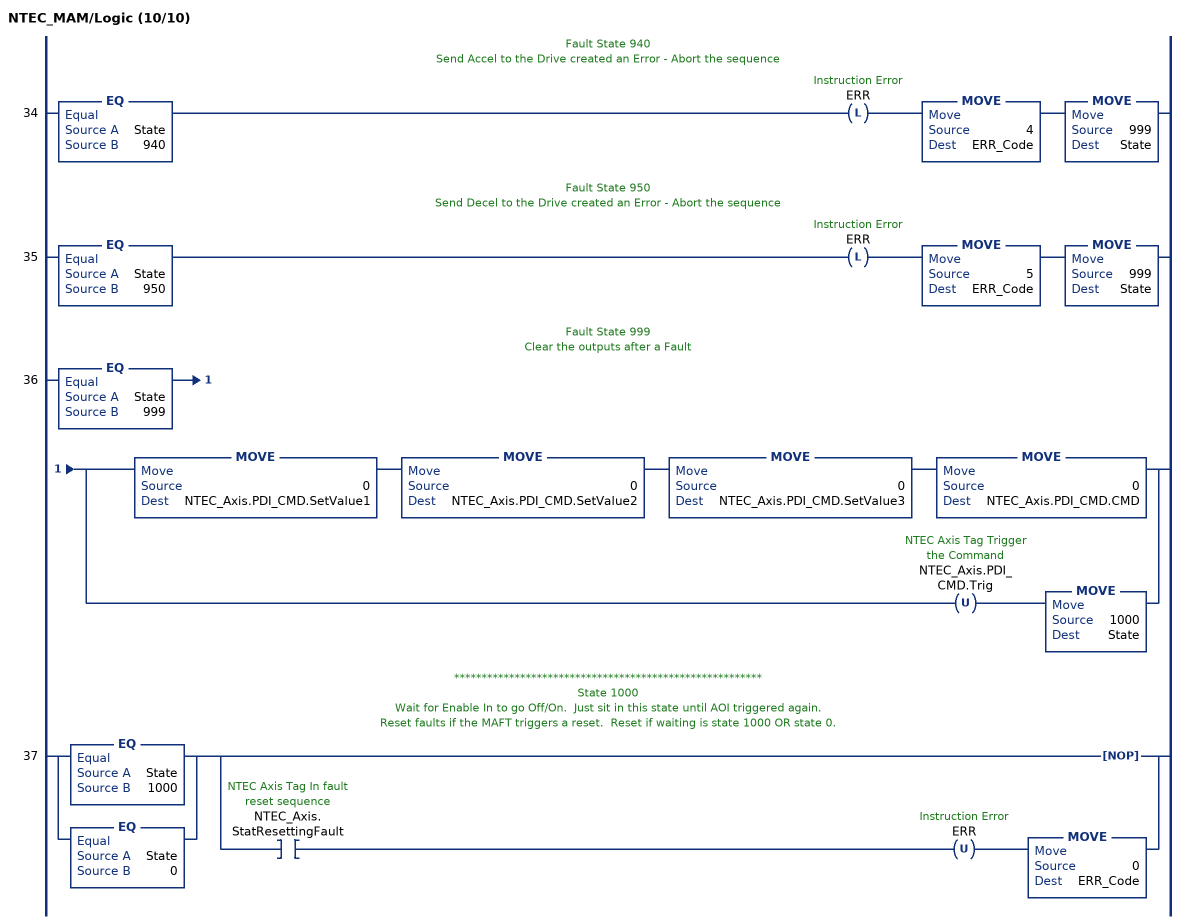
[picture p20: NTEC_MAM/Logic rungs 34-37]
   // Fault State 940
   // Send Accel to the Drive created an Error - Abort the sequence
   34: EQ(State,940)OTL(ERR)MOVE(4,ERR_Code)MOVE(999,State);
   // Fault State 950
   // Send Decel to the Drive created an Error - Abort the sequence
   35: EQ(State,950)OTL(ERR)MOVE(5,ERR_Code)MOVE(999,State);
   // Fault State 999
   // Clear the outputs after a Fault
   36: EQ(State,999)[MOVE(0,NTEC_Axis.PDI_CMD.SetValue1) MOVE(0,NTEC_Axis.PDI_CMD.SetValue2) MOVE(0,NTEC_Axis.PDI_CMD.SetValue3) MOVE(0,NTEC_Axis.PDI_CMD.CMD) ,OTU(NTEC_Axis.PDI_CMD.Trig) MOVE(1000,State) ];
   // ********************************************************
   // State 1000
   // Wait for Enable In to go Off/On.  Just sit in this state until AOI triggered again.
   // Reset faults if the MAFT triggers a reset.  Reset if waiting is state 1000 OR state 0.
   37: [EQ(State,1000) ,EQ(State,0) ][NOP() ,XIC(NTEC_Axis.StatResettingFault) OTU(ERR) MOVE(0,ERR_Code) ];
END_ROUTINE

ROUTINE Postscan   (* ladder *)
// Home Post-Scan Routine
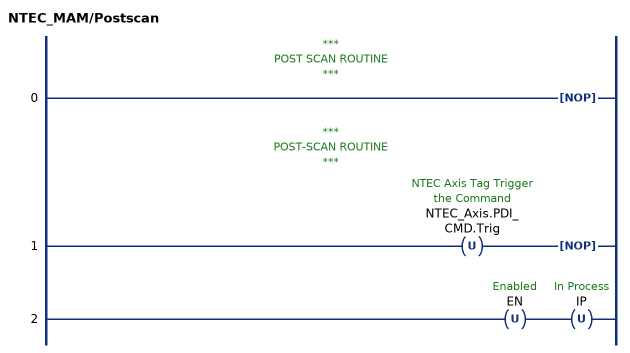
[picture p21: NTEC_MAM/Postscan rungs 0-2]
   // ***
   // POST SCAN ROUTINE
   // ***
   0: NOP();
   // ***
   // POST-SCAN ROUTINE
   // ***
   1: OTU(NTEC_Axis.PDI_CMD.Trig)NOP();
   2: OTU(EN)OTU(IP);
END_ROUTINE

ROUTINE Prescan   (* ladder *)
// Home Pre-Scan Routine
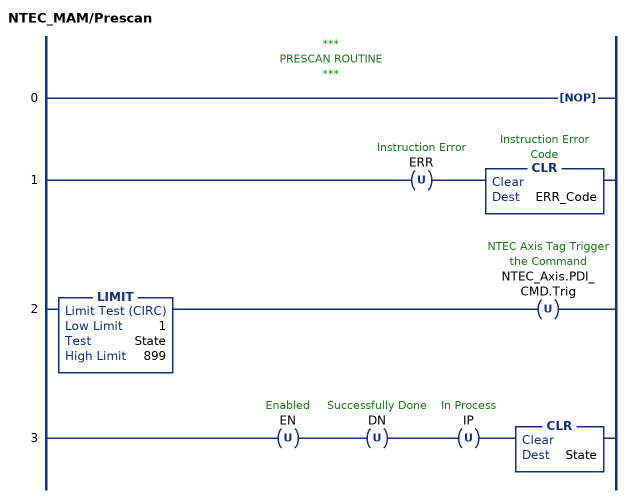
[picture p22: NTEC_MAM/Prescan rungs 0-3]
   // ***
   // PRESCAN ROUTINE
   // ***
   0: NOP();
   1: OTU(ERR)CLR(ERR_Code);
   2: LIMIT(1,State,899)OTU(NTEC_Axis.PDI_CMD.Trig);
   3: OTU(EN)OTU(DN)OTU(IP)CLR(State);
END_ROUTINE
END_ADD_ON_INSTRUCTION
